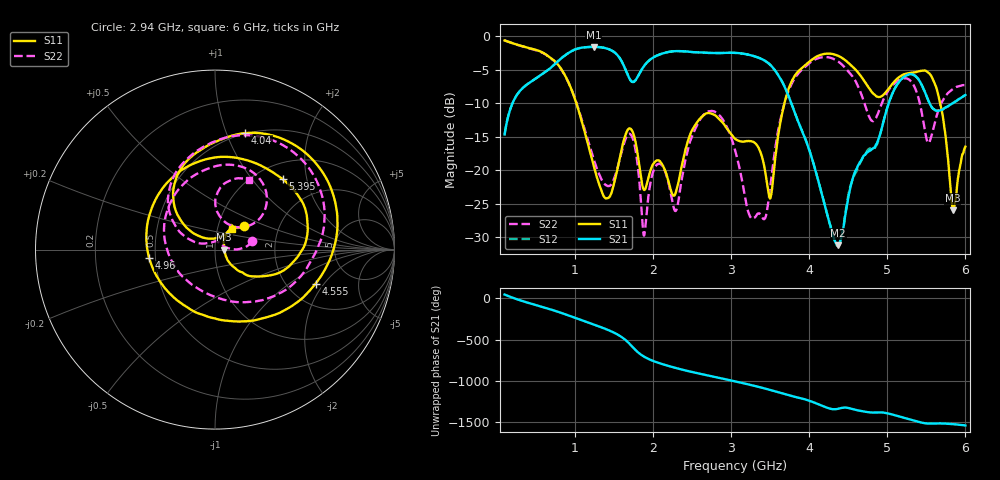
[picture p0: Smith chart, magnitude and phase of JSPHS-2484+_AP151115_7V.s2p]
!Mini-Circuits Laboratory
!S-Parameters
!Run/Lot/Date Code:MF33450/NA/1551
!Fixture/SN/Due: 90-4-20-21/70546/03/17/16
!Connection:PORT<IN> - pin<1>; PORT<OUT> - pin<7>;PORT<BIAS> - pin<4>;
!Tested With:PORT EXTENTION
!Network Analyzer:AG E5071C/74883/05/12/16
!Created: 01-07-2016 at 14:10:05
!MODEL: JSPHS-2484+
!S/N: V=7V
# MHZ S DB R 50
!Frequency  S11 dB  S11 DEG  S21 dB  S21 DEG  S12 dB  S12 DEG  S22 dB  S22 DEG
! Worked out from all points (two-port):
!   1181 points, 100 MHz to 6 GHz, reference 50 ohm
!   highest |S21| = -1.62 dB at 1.24 GHz (marker M1); lowest = -31.2 dB at 4.37 GHz (marker M2)
!   |S21| within 3 dB of the highest: 702.8 MHz to 1.634 GHz (931.4 MHz wide, 79.7 % of centre); 1.877 GHz to 3.528 GHz (1.652 GHz wide, 61.1 % of centre)
!   lowest |S11| = -25.9 dB at 5.84 GHz (marker M3), VSWR 1.11, Z = 55.3 + j0.00423 ohm
!   |S11| at or under -10 dB: 1.018 GHz to 3.683 GHz (2.665 GHz wide, 113 % of centre); 5.677 GHz to end of sweep
!   |S22| runs from -29.7 to -0.7 dB; largest |S21 - S12| = 0.0061
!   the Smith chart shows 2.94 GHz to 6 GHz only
!   S11 on the Smith chart (normalised r, x): 2.94 GHz: 1.32, +0.36; 4.04 GHz: 0.49, +1.17; 4.555 GHz: 2.84, -1.65; 4.96 GHz: 0.46, -0.05; 5.395 GHz: 1.29, +1.45; 6 GHz: 1.18, +0.28
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100  -0.66 -42.0  -14.65 47.7  -14.65 47.7  -0.66 -41.9
490  -2.02 -165.2  -6.40 -77.0  -6.40 -77.0  -2.06 -168.2
860  -5.59 89.2  -3.00 174.3  -3.00 174.3  -5.62 85.3
1085  -12.58 12.3  -1.74 97.2  -1.74 97.2  -12.36 8.1
1240  -19.27 -42.5  -1.62 45.0  -1.61 45.0  -18.30 -51.8
1530  -20.58 174.3  -2.67 -67.7  -2.67 -67.7  -20.30 -168.0
1675  -13.99 87.5  -5.74 -165.3  -5.74 -165.3  -14.73 103.0
1805  -17.70 18.1  -6.05 70.7  -6.05 70.7  -19.33 14.8
2070  -18.52 34.3  -2.81 -59.3  -2.81 -59.4  -19.03 43.4
2485  -14.38 78.8  -2.38 -166.6  -2.38 -166.6  -15.39 81.7
2940  -13.68 39.3  -2.50 100.1  -2.50 100.0  -13.41 12.7
3050  -15.29 44.6  -2.51 77.1  -2.51 77.1  -16.98 1.9
3430  -19.73 56.1  -3.66 -9.0  -3.66 -9.0  -27.21 111.9
4035  -3.51 76.1  -18.20 -169.3  -18.18 -169.5  -3.76 78.7
4040  -3.46 75.3  -18.40 -171.1  -18.39 -171.3  -3.72 77.8
4370  -2.95 17.9  -31.15 104.7  -31.29 104.9  -3.78 19.4
4555  -4.56 -18.6  -21.31 101.7  -21.38 99.2  -6.01 -17.3
4960  -8.65 -172.5  -12.35 57.4  -12.30 57.5  -9.21 139.6
5020  -7.79 156.0  -9.94 46.0  -9.93 45.9  -7.98 118.3
5395  -5.28 46.3  -6.37 -52.4  -6.38 -52.5  -9.05 38.3
5840  -25.94 0.0  -9.99 -80.8  -9.99 -80.9  -7.87 75.8
6000  -16.47 50.2  -8.78 -97.0  -8.79 -97.0  -7.30 63.9
